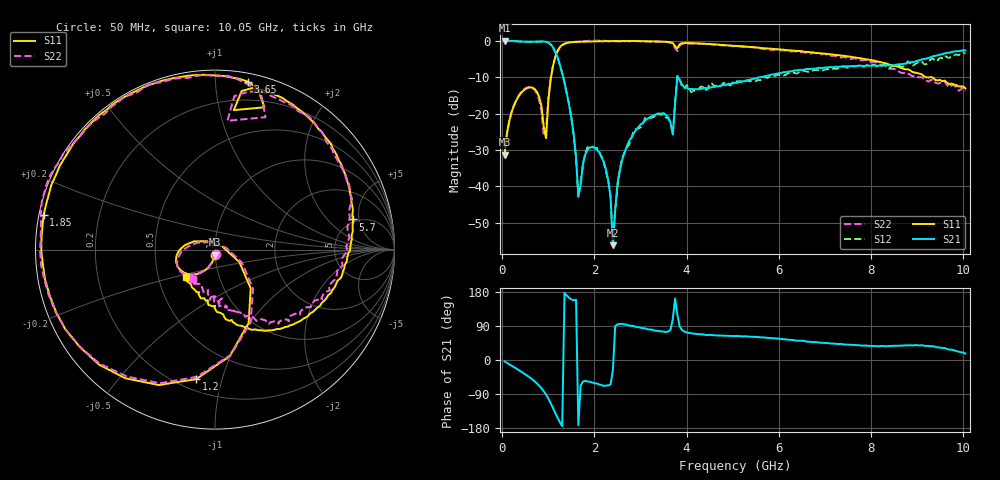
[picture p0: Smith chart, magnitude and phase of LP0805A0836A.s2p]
! AVX THIN FILM OPERATION
! 0805 Size Low Pass Filter P/N  LP0805A0836AWTR
! Network Analyzer HP8720ES.07.64: Feb 23, 2000 Serial No. US39172382
! Hewlett-Packard
! 2 Feb 2003  02:28:13
! Frequency  S11  S21  S12  S22
# HZ  S  DB R  50
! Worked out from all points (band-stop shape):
!   201 points, 50 MHz to 10.05 GHz, reference 50 ohm
!   highest |S21| = -0.03 dB at 50 MHz (marker M1); lowest = -56.2 dB at 2.4 GHz (marker M2)
!   |S21| within 3 dB of the highest: start of sweep to 1.152 GHz; 9.785 GHz to end of sweep
!   lowest |S11| = -31.3 dB at 50 MHz (marker M3), VSWR 1.06, Z = 50 - j2.73 ohm
!   |S11| at or under -10 dB: start of sweep to 1.059 GHz; 9.189 GHz to end of sweep
!   |S22| runs from -32.2 to 0.1 dB; largest |S21 - S12| = 0.15
!   S11 on the Smith chart (normalised r, x): 50 MHz: 1.00, -0.05; 1.2 GHz: 0.27, -0.83; 1.85 GHz: 0.01, +0.10; 3.65 GHz: 0.06, +1.21; 5.7 GHz: 4.66, +4.10; 10.05 GHz: 0.69, -0.22
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5e7  -31.27 -88.4  -0.03 -3.9  0.03 -3.8  -32.23 -72.6
2e8  -19.66 -109.8  -0.05 -15.0  -0.10 -14.9  -19.70 -110.4
5.5e8  -12.96 -150.3  -0.29 -42.0  -0.35 -42.3  -12.82 -148.4
9.5e8  -26.76 18.6  -0.32 -91.4  -0.32 -91.2  -24.20 10.2
1.2e9  -2.74 -98.3  -4.57 -152.6  -4.51 -152.4  -2.91 -98.0
1.5e9  -0.43 -158.4  -21.30 160.0  -21.34 157.6  -0.41 -158.6
1.65e9  -0.33 -174.9  -42.73 -172.2  -42.83 -168.5  -0.24 -175.0
1.75e9  -0.28 176.3  -33.86 -56.7  -34.09 -58.6  -0.24 176.0
1.85e9  -0.23 168.4  -29.97 -56.7  -29.26 -59.4  -0.07 168.2
2.25e9  -0.12 143.3  -35.40 -67.5  -36.12 -68.9  -0.09 144.9
2.35e9  -0.11 137.8  -43.18 -64.3  -42.67 -65.5  -0.15 139.1
2.4e9  -0.11 135.3  -56.23 -26.8  -56.42 -24.4  -0.13 136.2
2.6e9  -0.09 125.4  -32.77 95.2  -32.10 92.0  -0.15 125.8
3.4e9  -0.26 90.9  -20.01 76.1  -20.16 71.4  -0.28 90.2
3.65e9  -0.41 79.0  -22.50 79.7  -22.45 80.5  -0.57 78.1
3.7e9  -0.62 75.3  -25.79 107.8  -25.80 110.3  -0.86 73.6
3.8e9  -2.11 82.3  -9.70 119.2  -9.77 117.5  -2.84 84.5
5.05e9  -1.42 34.0  -11.58 63.0  -10.92 60.4  -1.49 32.9
5.7e9  -2.09 12.3  -9.74 59.2  -10.00 56.0  -2.26 13.4
6.75e9  -3.22 -20.6  -7.67 47.1  -8.15 47.0  -3.37 -19.5
8.4e9  -6.59 -67.8  -6.83 36.6  -7.66 31.2  -7.66 -61.6
1.005e10  -13.08 -136.5  -2.69 17.1  -3.59 14.3  -13.75 -126.6
